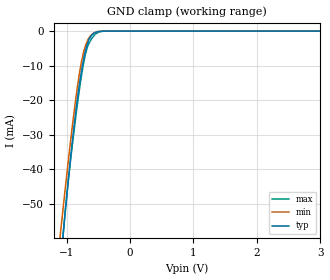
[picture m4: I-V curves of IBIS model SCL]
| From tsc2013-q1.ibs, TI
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|   1.8V SCL Model
[Model] SCL
Model_type Input
Vinl = 0.54
Vinh = 1.26
|   typ   min   max
|   (nom PVT)   (Fast PVT)   (Slow PVT)
C_comp   8.50433E-12   7.88656E-12   8.98759E-12
|Where nom PVT is NOM Process, 1.8V,27C
|   Fast PVT is Strong Process, 2.07V, -40C
|   Slow PVT is Weak Process, 1.53V, 85C
[Voltage Range]   1.8   1.62   1.98
[Temperature Range]   30   88   -40
[Power Clamp Reference]   1.8   1.62   1.98
[GND Clamp Reference]   0   0   0
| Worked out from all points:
|   GND clamp passes 1 mA (typ) near -0.59 V on its own axis
[GND Clamp]
|   Voltage   I(typ)   I(min)   I(max)
-1.8V     -218.2mA   -187.6mA   -259.9mA
-1.098V   -67.97mA   -58.97mA   -69.14mA
-1.058V   -60.04mA   -52.14mA   -59.92mA
-1.036V   -55.62mA   -48.32mA   -55.29mA
-977.2mV  -44.32mA   -38.52mA   -44.07mA
-909.2mV  -32.18mA   -27.67mA   -33.13mA
-787.7mV  -14.31mA   -11.24mA   -15.79mA
-731.2mV  -8.248mA   -6.097mA   -9.317mA
-680.7mV  -4.194mA   -3.294mA   -5.227mA
-570.6mV  -690.5uA   -526.5uA   -1.429mA
-418.1mV  -20.79uA   -22.21uA   -27uA
3.6V      0A         0A         0A
[POWER Clamp]
|   SCR cell for ESD function. Effects occurr above VDD x 2
|   Voltage   I(typ)   I(min)   I(max)
-1.8V     0A         0A         0A
0V        0A         0A         0A
3.6V      0A         0A         0A
